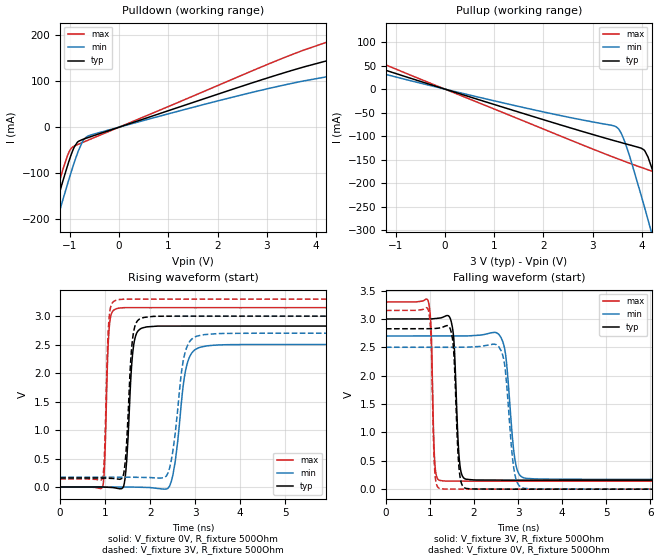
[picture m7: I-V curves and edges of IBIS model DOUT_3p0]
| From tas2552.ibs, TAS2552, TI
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|   Model
[Model]   DOUT_3p0
Model_type   Output
Polarity   Non-Inverting
Vmeas = 1.5
Vref = 0
Cref = 1pF
Rref = 1000000
|   typ   min   max
C_comp   1.241pF   1.153pF   1.378pF
[Voltage Range]   3   2.7   3.3
[Temperature Range]   27   125   -40
[Pullup Reference]   3   2.7   3.3
[Pulldown Reference]   -0   -0   -0
[Power Clamp Reference]   3   2.7   3.3
[GND Clamp Reference]   -0   -0   -0
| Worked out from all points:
|   slope of the pulldown table from 0 to 0.45 V, typ, clamps not added: 27.9 ohm
|   slope of the pullup table from 0 to 0.45 V, typ, clamps not added: 30.6 ohm
|   falling waveform, V_fixture 3V, R_fixture 500Ohm: 20-80 % time 90.3ps typ, 160ps min, 58.3ps max; typ from 3 V to 0.158 V
|   rising waveform, V_fixture 0V, R_fixture 500Ohm: 20-80 % time 115ps typ, 211ps min, 70.5ps max; typ from 0 V to 2.83 V
|   rising waveform, V_fixture 3V, R_fixture 500Ohm: 20-80 % time 115ps typ, 218ps min, 70ps max; typ from 0.158 V to 3 V
|   falling waveform, V_fixture 0V, R_fixture 500Ohm: 20-80 % time 90.1ps typ, 158ps min, 58.2ps max; typ from 2.83 V to 0 V
[Pulldown]
|   Voltage   I(typ)   I(min)   I(max)
-3V       -852.8mA   -882.8mA   -835.9mA
-1.686V   -326mA     -364.1mA   -302.6mA
-1.362V   -199.3mA   -239.4mA   -174.3mA
-1.308V   -178.6mA   -219mA     -153.4mA
-1.047V   -82.8mA    -122.7mA   -60.97mA
-912mV    -42.99mA   -76.59mA   -41.14mA
-750mV    -27.03mA   -32.47mA   -33.66mA
-588mV    -21.11mA   -17.5mA    -26.36mA
3.768V    131.5mA    100.9mA    168.4mA
4.911V    161.8mA    120.8mA    206.4mA
5.442V    172.1mA    126.7mA    218mA
5.991V    180.2mA    130.9mA    225.8mA
[Pullup]
|   Voltage   I(typ)   I(min)   I(max)
-3V       100.4mA    79.08mA    129.7mA
3.453V    -109.8mA   -78.78mA   -145.6mA
3.543V    -112.4mA   -86.6mA    -149.2mA
3.651V    -115.6mA   -110.8mA   -153.5mA
4.038V    -128.5mA   -244mA     -168.1mA
4.128V    -144.4mA   -277.7mA   -171.4mA
4.227V    -174.3mA   -315.3mA   -174.9mA
4.524V    -283.2mA   -429.6mA   -185.5mA
4.569V    -300.5mA   -447.1mA   -189.6mA
4.767V    -377.6mA   -524.4mA   -248mA
4.983V    -462.9mA   -609.2mA   -330.2mA
5.991V    -866.6mA   -1.008A    -735.2mA
[Ramp]
R_load = 500
|   typ   min   max
dV/dt_r   1.69648/1.15177e-10   1.50106/2.11393e-10   1.89049/7.0541e-11
dV/dt_f   1.70491/9.02891e-11   1.51629/1.59638e-10   1.89533/5.82721e-11
[Falling Waveform]
V_fixture = 3V
V_fixture_min = 2.7V
V_fixture_max = 3.3V
R_fixture = 500Ohm
C_fixture = 0F
|   Time   V(typ)   V(min)   V(max)
0s        3V         2.7V       3.3V
956.9ps   3.001V     2.701V     3.32V
1.119ns   3.008V     2.701V     372.4mV
1.314ns   3.039V     2.702V     144.7mV
1.699ns   320.7mV    2.702V     142mV
1.986ns   163.2mV    2.708V     141.1mV
2.647ns   159.6mV    2.61V      141.1mV
2.953ns   158.6mV    417.9mV    141.1mV
3.376ns   158.5mV    181.4mV    141.1mV
100ns     158.5mV    172.8mV    141.1mV
[Rising Waveform]
V_fixture = 0V
V_fixture_min = 0V
V_fixture_max = 0V
R_fixture = 500Ohm
C_fixture = 0F
|   Time   V(typ)   V(min)   V(max)
0s        723.9pV    16.8nV     330.7pV
948.1ps   -643.6uV   -905.1nV   15.73mV
1.098ns   -6.505mV   -1.051uV   2.86V
1.422ns   50.21mV    -1.366uV   3.149V
1.651ns   2.568V     -2.073mV   3.149V
2.168ns   2.826V     -25.24mV   3.149V
2.506ns   2.826V     210.7mV    3.149V
2.868ns   2.826V     2.269V     3.149V
3.649ns   2.826V     2.498V     3.149V
100ns     2.827V     2.502V     3.151V
[Rising Waveform]
V_fixture = 3V
V_fixture_min = 2.7V
V_fixture_max = 3.3V
R_fixture = 500Ohm
C_fixture = 0F
|   Time   V(typ)   V(min)   V(max)
0s        158.5mV    172.8mV    141.1mV
934.7ps   157.6mV    172.5mV    143.4mV
1.098ns   152.7mV    172.4mV    3.046V
1.422ns   278.6mV    172.3mV    3.298V
1.637ns   2.739V     171mV      3.298V
2.068ns   2.996V     162.7mV    3.298V
2.433ns   3V         334.8mV    3.298V
2.84ns    3V         2.501V     3.298V
3.499ns   3V         2.693V     3.298V
100ns     3V         2.7V       3.3V
[Falling Waveform]
|Gnd
V_fixture = 0V
V_fixture_min = 0V
V_fixture_max = 0V
R_fixture = 500Ohm
C_fixture = 0F
|   Time   V(typ)   V(min)   V(max)
0s        2.827V     2.502V     3.151V
956.9ps   2.829V     2.501V     3.166V
1.119ns   2.834V     2.501V     220mV
1.314ns   2.864V     2.501V     2.934mV
1.682ns   212.6mV    2.502V     834.1uV
1.919ns   4.884mV    2.506V     -22.54uV
2.612ns   1.216mV    2.445V     -25.7uV
2.925ns   173.3uV    264.3mV    -25.62uV
3.278ns   -21.3uV    6.235mV    -25.53uV
100ns     729.1pV    16.81nV    330.7pV
